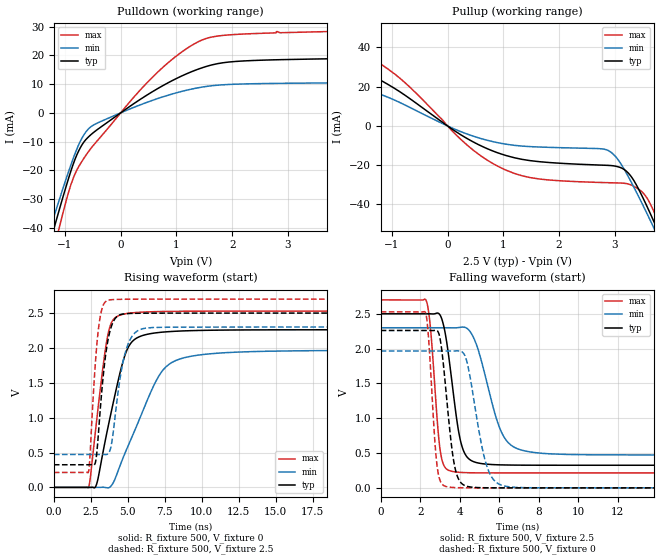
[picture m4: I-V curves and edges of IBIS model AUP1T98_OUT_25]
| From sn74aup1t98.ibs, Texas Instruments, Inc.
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[Model]   AUP1T98_OUT_25
Model_type  Output
Vref =   0
Rref =   1E6
Cref =   30p
Vmeas =   1.25
| variable   typ   min   max
C_comp   2.77pF   1.87pF   4.14pF
| C_pullup   3.12pF   1.87pF   4.14pF
| C_pulldown   2.42pF   2.13pF   2.99pF
[Temperature Range]   40   100   -40
| Ambient temperature   25   85   -40
[Voltage range]   2.5   2.3   2.7
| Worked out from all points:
|   slope of the pulldown table from 0 to 0.375 V, typ, clamps not added: 75.2 ohm
|   slope of the pullup table from 0 to 0.375 V, typ, clamps not added: 55.1 ohm
|   rising waveform, R_fixture 500, V_fixture 0: 20-80 % time 1.4ns typ, 2.41ns min, 859ps max; typ from 0 V to 2.26 V
|   falling waveform, R_fixture 500, V_fixture 2.5: 20-80 % time 621ps typ, 1.07ns min, 391ps max; typ from 2.5 V to 0.325 V
|   rising waveform, R_fixture 500, V_fixture 2.5: 20-80 % time 611ps typ, 792ps min, 469ps max; typ from 0.325 V to 2.5 V
|   falling waveform, R_fixture 500, V_fixture 0: 20-80 % time 498ps typ, 751ps min, 332ps max; typ from 2.26 V to 0 V
[Pulldown]
| AUP1T98_OUT_25
|   Voltage   I(typ)   I(min)   I(max)
-3.6V     -214mA     -193.5mA   -239.7mA
-1.26V    -44.55mA   -39.92mA   -52.42mA
-1.205V   -40.74mA   -36.52mA   -48.02mA
-1.115V   -34.57mA   -31.02mA   -40.91mA
-800mV    -15.22mA   -13.22mA   -20.4mA
-685mV    -10.84mA   -8.445mA   -16.54mA
-540mV    -7.689mA   -4.911mA   -12.5mA
675mV     8.558mA    5.038mA    14.35mA
1.105V    12.9mA     7.5mA      21.28mA
1.52V     16.03mA    9.129mA    25.76mA
2.585V    18.34mA    10.19mA    27.69mA
7.2V      19.61mA    10.73mA    29.61mA
[Pullup]
| AUP1T98_OUT_25
|   Voltage   I(typ)   I(min)   I(max)
-3.6V     37.28mA    23.5mA     50.35mA
-2.355V   24.65mA    15.21mA    35.57mA
-1.425V   26.01mA    17.2mA     35.58mA
-760mV    15.58mA    10.63mA    21.96mA
405mV     -7.279mA   -4.651mA   -11.04mA
1.05V     -15.07mA   -9.293mA   -22.54mA
2.845V    -20.04mA   -12.07mA   -28.88mA
3.17V     -22.17mA   -22.09mA   -29.2mA
3.455V    -33.67mA   -37.48mA   -32.73mA
3.685V    -47.61mA   -50.92mA   -42.5mA
3.82V     -56.28mA   -59.04mA   -51.47mA
7.2V      -294.7mA   -278.7mA   -311.5mA
[Ramp]
| AUP1T98_OUT_25
| variable   typ   min   max
dV/dt_r   1.36/1.41E-09   1.18/2.41E-09   1.52/8.61E-10
dV/dt_f   1.31/6.30E-10   1.10/1.07E-09   1.50/3.94E-10
R_load = 500
[Rising Waveform]
| AUP1T98_OUT_25
R_fixture =   500
C_fixture =   0
L_fixture =   0
V_fixture =   0
V_fixture_min = 0
V_fixture_max = 0
|   Time   V(typ)   V(min)   V(max)
0s        19.04nV    76.96nV    1.464nV
2.355ns   -15.1uV    26.89nV    5.199mV
2.885ns   42.15mV    -32.82uV   940.3mV
3.6ns     799.5mV    -5.486mV   2.128V
3.935ns   1.134V     37.89mV    2.378V
4.48ns    1.647V     313.5mV    2.471V
5.305ns   2.093V     734.8mV    2.503V
7.08ns    2.221V     1.59V      2.521V
8.82ns    2.245V     1.86V      2.526V
34.99ns   2.261V     1.966V     2.528V
[Falling Waveform]
| AUP1T98_OUT_25
R_fixture =   500
C_fixture =   0
L_fixture =   0
V_fixture =   2.5
V_fixture_min = 2.3
V_fixture_max = 2.7
|   Time   V(typ)   V(min)   V(max)
0s        2.5V       2.3V       2.7V
2.31ns    2.5V       2.3V       2.686V
2.52ns    2.5V       2.3V       2.293V
3.015ns   2.477V     2.3V       532.5mV
3.58ns    1.583V     2.299V     238.9mV
3.985ns   747.8mV    2.304V     223.1mV
4.375ns   441.4mV    2.29V      218mV
6.12ns    329.9mV    795.3mV    214.5mV
7.34ns    325.9mV    527.9mV    214.4mV
34.99ns   324.7mV    472mV      214.4mV
[Rising Waveform]
| AUP1T98_OUT_25
R_fixture =   500
C_fixture =   0
L_fixture =   0
V_fixture =   2.5
V_fixture_min = 2.3
V_fixture_max = 2.7
|   Time   V(typ)   V(min)   V(max)
0s        324.7mV    472mV      214.4mV
2.345ns   324.7mV    472mV      223.7mV
2.8ns     347.7mV    472mV      1.756V
3ns       730.9mV    471.9mV    2.241V
3.345ns   1.611V     473mV      2.615V
3.665ns   2.117V     481.9mV    2.683V
3.91ns    2.321V     635.1mV    2.692V
4.82ns    2.49V      1.923V     2.698V
5.98ns    2.498V     2.274V     2.699V
34.99ns   2.5V       2.3V       2.7V
[Falling Waveform]
| AUP1T98_OUT_25
R_fixture =   500
C_fixture =   0
L_fixture =   0
V_fixture =   0
V_fixture_min = 0
V_fixture_max = 0
|   Time   V(typ)   V(min)   V(max)
0s        2.261V     1.966V     2.528V
2.275ns   2.261V     1.966V     2.51V
2.845ns   2.26V      1.966V     335.8mV
3.32ns    1.342V     1.966V     17.9mV
3.665ns   438.4mV    1.966V     5.443mV
3.985ns   102.8mV    1.966V     1.991mV
4.385ns   20.77mV    1.788V     604.1uV
5.38ns    1.309mV    304.7mV    52.34uV
6.29ns    218.9uV    23.99mV    9.004uV
34.99ns   17nV       65.86nV    -18.84nV
